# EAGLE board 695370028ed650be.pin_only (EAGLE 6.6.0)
REV: D

Size 15.24 x 26.67 mm. Coordinates in mm from the lower left corner, seen from the top.
Outline: 15.24,25.4 15.24,2.29 14.48,1.52 11.18,1.52 9.65,0 2.54,0 0.76,1.78 0,1.78 0,25.4 arc-90 1.27,26.67 4.83,26.67 5.21,26.29 10.03,26.29 10.41,26.67 13.97,26.67 arc-90 15.24,25.4
Copper layers (1*16): Top 0.035mm / dielectric 1.5mm / Bottom 0.035mm
Design rules "adafruit *": minimum track width 8mil, minimum drill 15.5mil, track to track 8mil, track to pad 8mil, pad to pad 8mil, via to via 8mil, smd to smd 8mil, copper to edge 10mil, drill to drill 8mil, minimum pad ring 10mil, minimum via ring 8mil, stop-mask expansion 2mil, vias tented up to drill 20mil, thermal gap 10mil
Net classes: 1 power: width 0.305 mm
Holes 2.2 mm at 1.52,20.19 13.72,20.19

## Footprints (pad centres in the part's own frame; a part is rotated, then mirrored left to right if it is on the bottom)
JSTPH2 = smd 1 x 4.6: 1 -1,-3.7; 2 1,-3.7 | smd 1.6 x 3.4: NC1 -3.4,1.5; NC2 3.4,1.5
0805-NO = smd 1.24 x 1.5: 1 -0.95,0; 2 0.95,0
0603-NO = smd 1.075 x 1: 1 -0.85,0; 2 0.85,0
4UCONN_20329_V2 = smd 1 x 2: BASE@1 -0.75,-2; BASE@2 0.75,-2 | smd 0.4 x 1.35: D+ 0,0.775; D- -0.65,0.775; GND 1.3,0.775; ID 0.65,0.775; VBUS -1.3,0.775 | drill 0.8 pad 1.143 offset: SPRT@1 -3.3,0.9; SPRT@2 3.3,0.9 | drill 0.9 pad 2.413 square: SPRT@3 -3.6,-1.9; SPRT@4 3.6,-1.9 | hole 0.7: -1.95,0; 1.95,0
SOD-123FL = smd 0.91 x 1.22: A 1.637,0; C -1.637,0
QFN32_5MM = smd 0.8 x 0.25: 1 -2.5,1.75; 2 -2.5,1.25; 3 -2.5,0.75; 4 -2.5,0.25; 5 -2.5,-0.25; 6 -2.5,-0.75; 7 -2.5,-1.25; 8 -2.5,-1.75; 17 2.5,-1.75; 18 2.5,-1.25; 19 2.5,-0.75; 20 2.5,-0.25; 21 2.5,0.25; 22 2.5,0.75; 23 2.5,1.25; 24 2.5,1.75 | smd 0.25 x 0.8: 9 -1.75,-2.5; 10 -1.25,-2.5; 11 -0.75,-2.5; 12 -0.25,-2.5; 13 0.25,-2.5; 14 0.75,-2.5; 15 1.25,-2.5; 16 1.75,-2.5; 25 1.75,2.5; 26 1.25,2.5; 27 0.75,2.5; 28 0.25,2.5; 29 -0.25,2.5; 30 -0.75,2.5; 31 -1.25,2.5; 32 -1.75,2.5 | smd 3.5 x 3.5: 33 0,0
1X05_ROUND_76 = drill 1 pad 1.93: 1 -5.08,0; 2 -2.54,0; 3 0,0; 4 2.54,0; 5 5.08,0
CHIPLED_0603_NOOUTLINE = smd 0.8 x 0.8: A 0,-0.75; C 0,0.75
APA102_2020 = smd 0.7 x 0.35: 1 -0.95,-0.75; 2 -0.95,0; 3 -0.95,0.75; 4 0.95,0.75; 5 0.95,0; 6 0.95,-0.75
BTN_KMR2_4.6X2.8 = smd 0.9 x 0.9: A 2.05,0.8; A' -2.05,0.8; B 2.05,-0.8; B' -2.05,-0.8
B1,27 = smd 1.27 x 1.27: TP 0,0
SOT23-5 = smd 0.55 x 1.2: 1 -0.95,-1.3; 2 0,-1.3; 3 0.95,-1.3; 4 0.95,1.3; 5 -0.95,1.3
FIDUCIAL_1MM = smd 1 x 1: 1 0,0
MOUNTINGHOLE_2.0_PLATED = drill 2.2 pad 3: P$1 0,0

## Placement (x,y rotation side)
BAT  JST-2PH  [JSTPH2]  7.62,22.99 0 bottom
C1  10uF  [0805-NO]  9.65,6.79 270 top
C2  1uF  [0603-NO]  4.06,15.3 270 top
C3  1uF  [0603-NO]  4.06,18.35 90 top
C8  10uF  [0805-NO]  10.35,3.37 270 top
CN1  4U#20329  [4UCONN_20329_V2]  7.62,22.35 180 top
D2  SCHOTTKY  [SOD-123FL]  9.86,9.33 0 top
D3  SCHOTTKY  [SOD-123FL]  5.46,9.33 180 top
IC3  ATSAMD21E  [QFN32_5MM]  8.69,17 90 top
JP3  [1X05_ROUND_76]  1.3,12.7 270 top
JP4  [1X05_ROUND_76]  13.97,12.7 90 top
L  red  [CHIPLED_0603_NOOUTLINE]  13.14,24.26 180 top
LED1  AP102-2020  [APA102_2020]  6.12,12.37 90 top
PWR  green  [CHIPLED_0603_NOOUTLINE]  2.1,24.26 180 top
Q2  reset  [BTN_KMR2_4.6X2.8]  6.73,3.17 0 top
R1  1.5K  [0603-NO]  14.35,24.1 270 top
R4  10K  [0603-NO]  0.89,24.13 270 top
SWC  TPB1,27  [B1,27]  4.25,16.41 0 bottom
SWD  TPB1,27  [B1,27]  4.25,14.41 0 bottom
U1  AP2112K-3.3  [SOT23-5]  6.03,6.6 270 top
U$1  [TRINKET_M0_BOTTOM]  15.24,0 0 bottom
U$6  FIDUCIAL_1MM  [FIDUCIAL_1MM]  6.41,3.05 0 top
U$8  MOUNTINGHOLE2.0  [MOUNTINGHOLE_2.0_PLATED]  1.91,3.81 0 top
U$9  MOUNTINGHOLE2.0  [MOUNTINGHOLE_2.0_PLATED]  13.34,3.81 0 top
U$12  [PCBFEAT-REV-040]  6.22,15.62 90 bottom
U$20  [TRINKET_M0_TOP]  0,0 0 top

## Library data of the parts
BAT C1-C3 C8 CN1 IC3 JP3 JP4 L LED1 PWR Q2 R1 R4 U1 U$12 = microbuilder
D2 D3 = adafruit
SWC SWD = testpad
U$1 U$20 = silks
U$6 U$8 U$9 = microbuilder; BOM: EXCLUDE

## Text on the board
bPlace: + | -
tDocu: D0/A4/SDA | D4/A2/RXD/MOSI | D1/A0/VOUT | D3/A3/TXD/SCK | D2/A1/SCL/MISO

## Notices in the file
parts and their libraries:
microbuilder: This work is placed in the public domain, and may be freely used for commercial and non-commercial work with the following conditions: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
